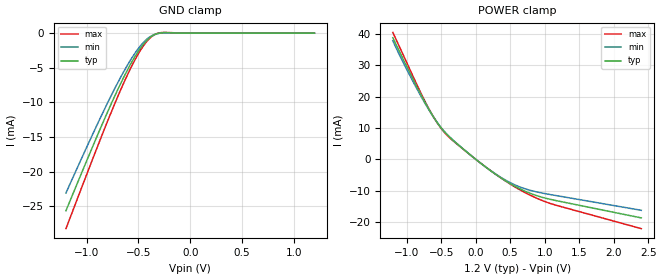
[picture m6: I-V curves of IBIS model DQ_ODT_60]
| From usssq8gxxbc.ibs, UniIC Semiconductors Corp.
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|   Model DQ_ODT_60
[Model] DQ_ODT_60
Model_type Input
Polarity   Non-Inverting
Enable   Active-High
Vinl =  8.300E-01
Vinh =  9.700E-01
C_comp   7.011E-13   7.005E-13   7.034E-13
C_comp_power_clamp   2.848E-13   2.839E-13   2.872E-13
C_comp_gnd_clamp   4.001E-13   3.984E-13   4.040E-13
[Model Spec]
Vinh   9.700E-01   9.250E-01   1.015E+00
Vinl   8.300E-01   7.850E-01   8.750E-01
[Temperature Range]   4.500E+01   9.500E+01   0.000E+00
[Voltage Range]   1.200E+00   1.140E+00   1.260E+00
[C Comp Corner]
C_comp_power_clamp   2.848E-13   2.872E-13   2.839E-13
C_comp_gnd_clamp   4.001E-13   3.984E-13   4.040E-13
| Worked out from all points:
|   GND clamp passes 1 mA (typ) near -0.42 V on its own axis
|   POWER clamp passes 1 mA (typ) near -0.06 V on its own axis
[GND_clamp]
|Voltage   I(typ)   I(min)   I(max)
-1.2V     -25.65mA   -23.09mA   -28.23mA
-875mV    -14.03mA   -12.46mA   -15.61mA
-750mV    -9.779mA   -8.622mA   -10.95mA
-650mV    -6.606mA   -5.771mA   -7.455mA
-575mV    -4.45mA    -3.844mA   -5.055mA
-500mV    -2.582mA   -2.194mA   -2.95mA
-425mV    -1.13mA    -939.9uA   -1.294mA
-375mV    -471.9uA   -392.7uA   -527.1uA
-325mV    -95.77uA   -92.13uA   -72.9uA
-250mV    61.16uA    36.38uA    113.9uA
-25mV     0A         0A         0A
1.2V      0A         0A         0A
[POWER_clamp]
|Voltage   I(typ)   I(min)   I(max)
-1.2V     38.8mA     37.84mA    40.49mA
-1.025V   30.83mA    29.78mA    32.13mA
-800mV    20.89mA    20.43mA    21.43mA
-650mV    14.91mA    14.79mA    14.99mA
-525mV    10.75mA    10.78mA    10.58mA
-425mV    8.103mA    8.181mA    7.882mA
-325mV    6.004mA    6.064mA    5.825mA
250mV     -4.195mA   -4.125mA   -4.174mA
575mV     -8.709mA   -8.253mA   -8.922mA
925mV     -11.9mA    -10.61mA   -12.83mA
1.15V     -13.13mA   -11.54mA   -14.59mA
2.4V      -18.73mA   -16.3mA    -22.16mA
